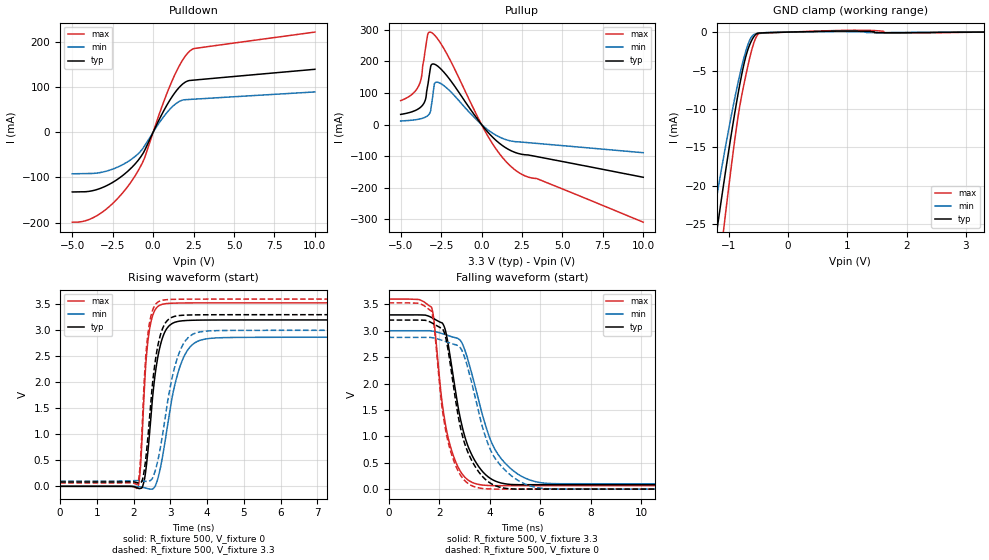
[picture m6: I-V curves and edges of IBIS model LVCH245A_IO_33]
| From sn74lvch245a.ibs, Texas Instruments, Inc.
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[Model]   LVCH245A_IO_33
Model_type  I/O
Vinl=0.8
Vinh=2.0
Enable   Active-Low
Vref =   0
Rref =   500
Cref =   50p
Vmeas =   1.5
| variable   typ   min   max
C_comp   4.45pF   4.03pF   5.66pF
| C_pullup   6.34pF   4.72pF   7.85pF
| C_pulldown   5.25pF   3.53pF   6.99pF
| C_tri-state   4.45pF   4.03pF   5.66pF
[Temperature Range]   40   100   -40
| Ambient temperature   25   85   -40
[Voltage range]   3.3   3   3.6
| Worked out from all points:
|   slope of the pulldown table from 0 to 0.495 V, typ, clamps not added: 13.6 ohm
|   slope of the pullup table from 0 to 0.495 V, typ, clamps not added: 16.5 ohm
|   GND clamp passes 1 mA (typ) near -0.61 V on its own axis
|   rising waveform, R_fixture 500, V_fixture 0: 20-80 % time 295ps typ, 469ps min, 181ps max; typ from 0 V to 3.2 V
|   falling waveform, R_fixture 500, V_fixture 3.3: 20-80 % time 828ps typ, 1.14ns min, 607ps max; typ from 3.3 V to 0.083 V
|   rising waveform, R_fixture 500, V_fixture 3.3: 20-80 % time 287ps typ, 459ps min, 176ps max; typ from 0.083 V to 3.3 V
|   falling waveform, R_fixture 500, V_fixture 0: 20-80 % time 811ps typ, 1.09ns min, 603ps max; typ from 3.2 V to 0 V
[GND Clamp]
| LVCH245A_IO_33
|   Voltage   I(typ)   I(min)   I(max)
-5V       -263.7mA   -222mA     -331.2mA
-1.295V   -31.01mA   -25.61mA   -39.85mA
-1.21V    -26.35mA   -21.72mA   -33.99mA
-1.17V    -24.2mA    -19.92mA   -31.27mA
-1.09V    -19.98mA   -16.41mA   -25.94mA
-1.055V   -18.17mA   -14.91mA   -23.66mA
-855mV    -8.564mA   -6.992mA   -11.62mA
-740mV    -4.041mA   -3.231mA   -6.652mA
-625mV    -1.263mA   -723.9uA   -2.69mA
-500mV    -133.9uA   -146.5uA   -238.3uA
1.11V     132.7uA    59.83uA    238.3uA
3.3V      26.32pA    97.07nA    -1.113uA
[Pulldown]
| LVCH245A_IO_33
|   Voltage   I(typ)   I(min)   I(max)
-5V       -132mA     -91.82mA   -198.7mA
-4.12V    -131.2mA   -91.3mA    -194.8mA
-3.21V    -123.3mA   -88.68mA   -178.2mA
-2.24V    -104.9mA   -77.74mA   -148mA
-1.33V    -78.13mA   -59.41mA   -108mA
-550mV    -41.86mA   -31.21mA   -58.49mA
450mV     33.38mA    24.55mA    47.28mA
1.11V     75.1mA     53.59mA    108.4mA
1.755V    104.2mA    70.16mA    155.4mA
2.31V     114.4mA    72.49mA    180.5mA
2.575V    115.3mA    73.08mA    185.1mA
10V       139mA      89mA       221.2mA
[Pullup]
| LVCH245A_IO_33
|   Voltage   I(typ)   I(min)   I(max)
-5V       32.03mA    11.21mA    75.69mA
-3.94V    48.46mA    16.28mA    117.2mA
-3.73V    56.47mA    18.6mA     145.9mA
-3.58V    65.86mA    20.98mA    200.7mA
-3.445V   83.4mA     24.02mA    248.1mA
-3.325V   123.8mA    28.1mA     285.2mA
-3.105V   188.8mA    58.74mA    291.4mA
-2.91V    190.9mA    129mA      283.3mA
-2.61V    180.5mA    132mA      263.6mA
350mV     -21.8mA    -15.16mA   -32.98mA
1.855V    -83.7mA    -52.55mA   -134.5mA
10V       -167mA     -89.26mA   -309.2mA
[Ramp]
| LVCH245A_IO_33
| variable   typ   min   max
dV/dt_r   1.94/3.03E-10   1.75/4.84E-10   2.14/1.86E-10
dV/dt_f   1.93/8.35E-10   1.74/1.15E-09   2.12/6.11E-10
R_load = 500
[Rising Waveform]
| LVCH245A_IO_33
R_fixture =   500
C_fixture =   0
L_fixture =   0
V_fixture =   0
V_fixture_min = 0
V_fixture_max = 0
|   Time   V(typ)   V(min)   V(max)
0s        280.2pV    4.034nV    33.78nV
2.105ns   -31.52mV   -4.244mV   -26.68mV
2.185ns   -40.97mV   -11.64mV   371.3mV
2.285ns   105.1mV    -25.1mV    1.782V
2.43ns    1.001V     -51.03mV   3.008V
2.64ns    2.413V     106.7mV    3.446V
2.9ns     3.032V     1.073V     3.514V
3.4ns     3.186V     2.538V     3.525V
4.245ns   3.198V     2.853V     3.527V
50ns      3.2V       2.866V     3.528V
[Falling Waveform]
| LVCH245A_IO_33
R_fixture =   500
C_fixture =   0
L_fixture =   0
V_fixture =   3.3
V_fixture_min = 3
V_fixture_max = 3.6
|   Time   V(typ)   V(min)   V(max)
0s        3.3V       3V         3.6V
1.695ns   3.252V     2.996V     3.449V
1.805ns   3.224V     2.987V     3.159V
2.155ns   3.126V     2.94V      1.516V
2.475ns   2.394V     2.89V      761.5mV
2.965ns   1.083V     2.701V     254mV
3.67ns    359.2mV    1.479V     78.97mV
4.61ns    100.4mV    490.9mV    64.39mV
6.3ns     83.02mV    107.1mV    64.99mV
50ns      83.11mV    100.9mV    64.84mV
[Rising Waveform]
| LVCH245A_IO_33
R_fixture =   500
C_fixture =   0
L_fixture =   0
V_fixture =   3.3
V_fixture_min = 3
V_fixture_max = 3.6
|   Time   V(typ)   V(min)   V(max)
0s        83.06mV    100.9mV    64.83mV
2.1ns     68.67mV    110.2mV    47.02mV
2.175ns   67.49mV    107.2mV    410.7mV
2.26ns    193.2mV    101.2mV    1.613V
2.415ns   1.17V      97.02mV    3.068V
2.61ns    2.512V     359mV      3.51V
2.86ns    3.137V     1.331V     3.586V
3.325ns   3.288V     2.702V     3.597V
4.075ns   3.298V     2.989V     3.599V
50ns      3.3V       3V         3.6V
[Falling Waveform]
| LVCH245A_IO_33
R_fixture =   500
C_fixture =   0
L_fixture =   0
V_fixture =   0
V_fixture_min = 0
V_fixture_max = 0
|   Time   V(typ)   V(min)   V(max)
0s        3.202V     2.874V     3.528V
1.695ns   3.153V     2.87V      3.373V
1.805ns   3.124V     2.861V     3.078V
2.15ns    3.025V     2.813V     1.431V
2.47ns    2.275V     2.761V     691.8mV
2.935ns   985.8mV    2.591V     203.2mV
3.695ns   248.9mV    1.207V     12.46mV
4.66ns    11.86mV    334.1mV    -339.6uV
6.34ns    15.91uV    3.71mV     166.9uV
50ns      47.73uV    89.04uV    15.6uV
